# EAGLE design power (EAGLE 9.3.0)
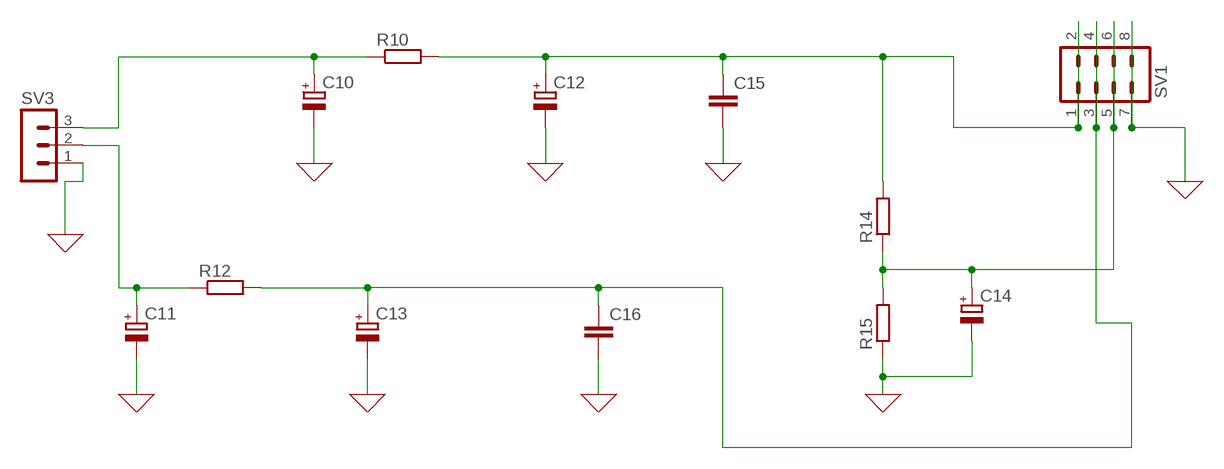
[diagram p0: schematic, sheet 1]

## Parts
C10  CPOL-EUB45181A  [B45181A]
C11  CPOL-EUB45181A  [B45181A]
C12  CPOL-EUB45181A  [B45181A]
C13  CPOL-EUB45181A  [B45181A]
C14  CPOL-EUB45181A  [B45181A]
C15  C-EUC0805  [C0805]
C16  C-EUC0805  [C0805]
R10  R-EU_M0805  [M0805]
R12  R-EU_M0805  [M0805]
R14  R-EU_M0805  [M0805]
R15  R-EU_M0805  [M0805]
SV1  MA04-2  [MA04-2]
SV3  MA03-1  [MA03-1]

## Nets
0: C10.- C11.- C12.- C13.- C14.- C15.2 C16.2 R15.1 SV1.7 SV1.8 SV3.1 ; supply symbol labelled GND
N$1: C10.+ R10.1 SV3.3
N$23: C12.+ C15.1 R10.2 R14.2 SV1.1 SV1.2
N$25: C11.+ R12.1 SV3.2
N$26: C13.+ C16.1 R12.2 SV1.3 SV1.4
N$28: C14.+ R14.1 R15.2 SV1.5 SV1.6

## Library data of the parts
C10-C14 = rcl:CPOL-EU: POLARIZED CAPACITOR, European symbol; SPICEPREFIX: C
C15 C16 = rcl:C-EU: CAPACITOR, European symbol; SPICEPREFIX: C
R10 R12 R14 R15 = rcl:R-EU_: RESISTOR, European symbol; SPICEPREFIX: R
SV1 = con-lstb:MA04-2: PIN HEADER; OC_FARNELL: unknown; OC_NEWARK: unknown
SV3 = con-lstb:MA03-1: PIN HEADER; OC_FARNELL: unknown; OC_NEWARK: unknown

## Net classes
0 default: width 0.305 mm, drill 0.406 mm, clearance 0.508 mm

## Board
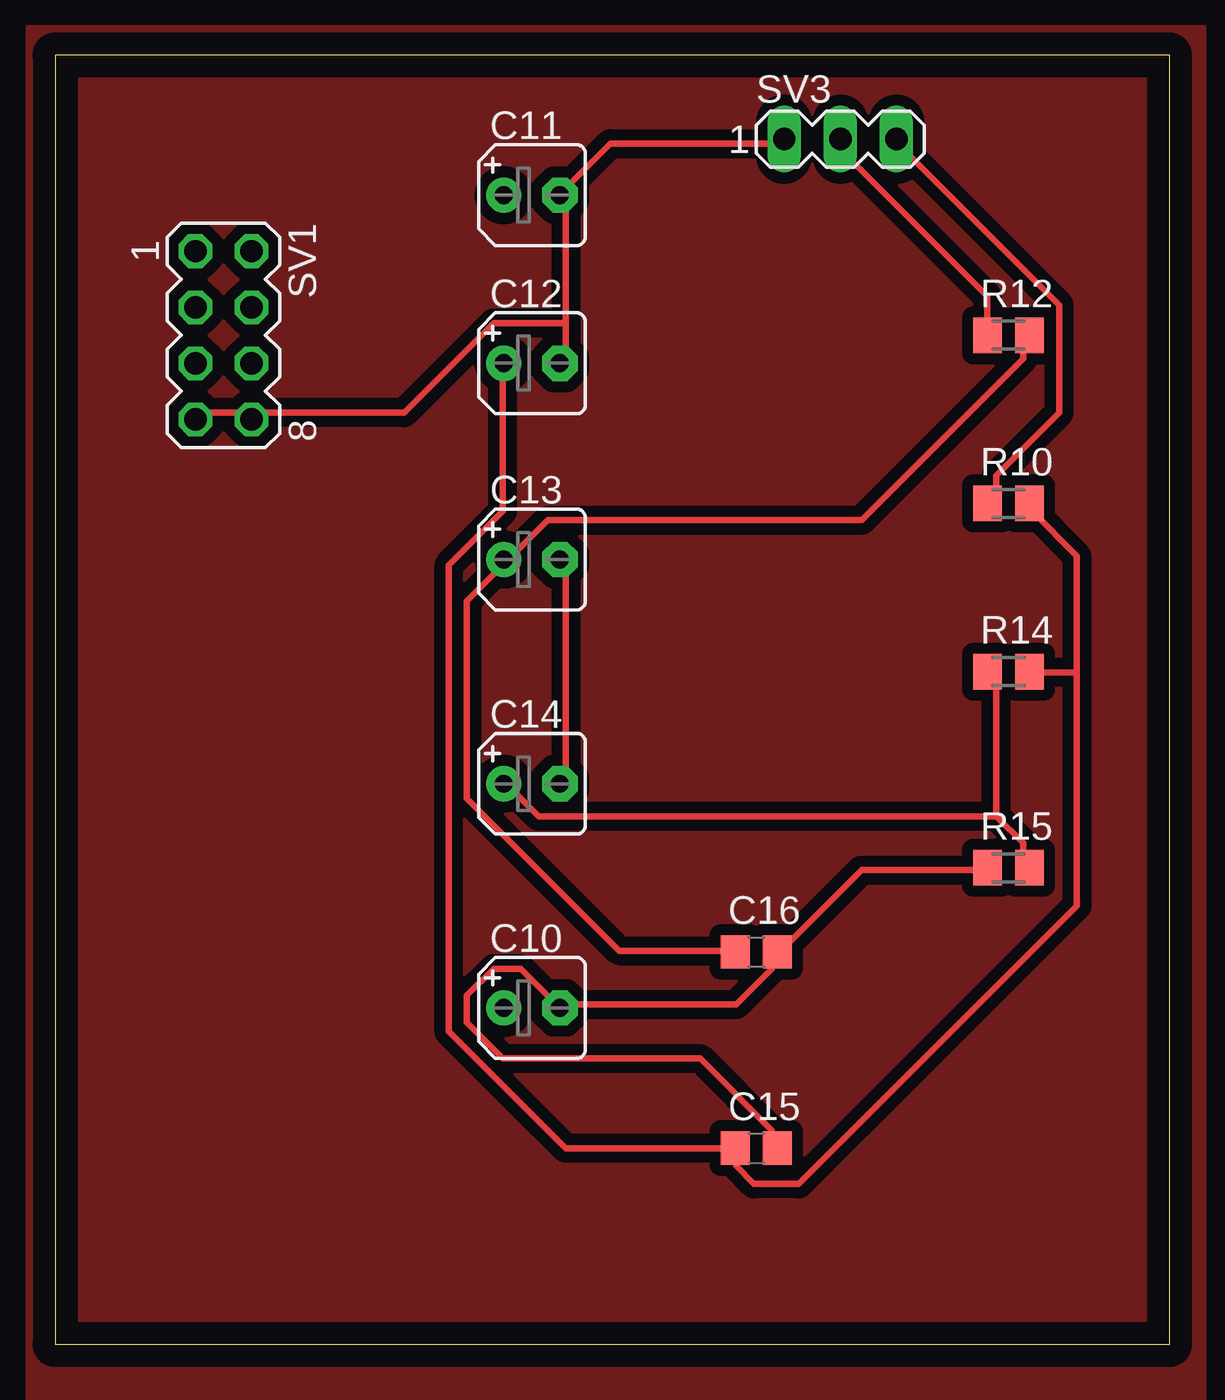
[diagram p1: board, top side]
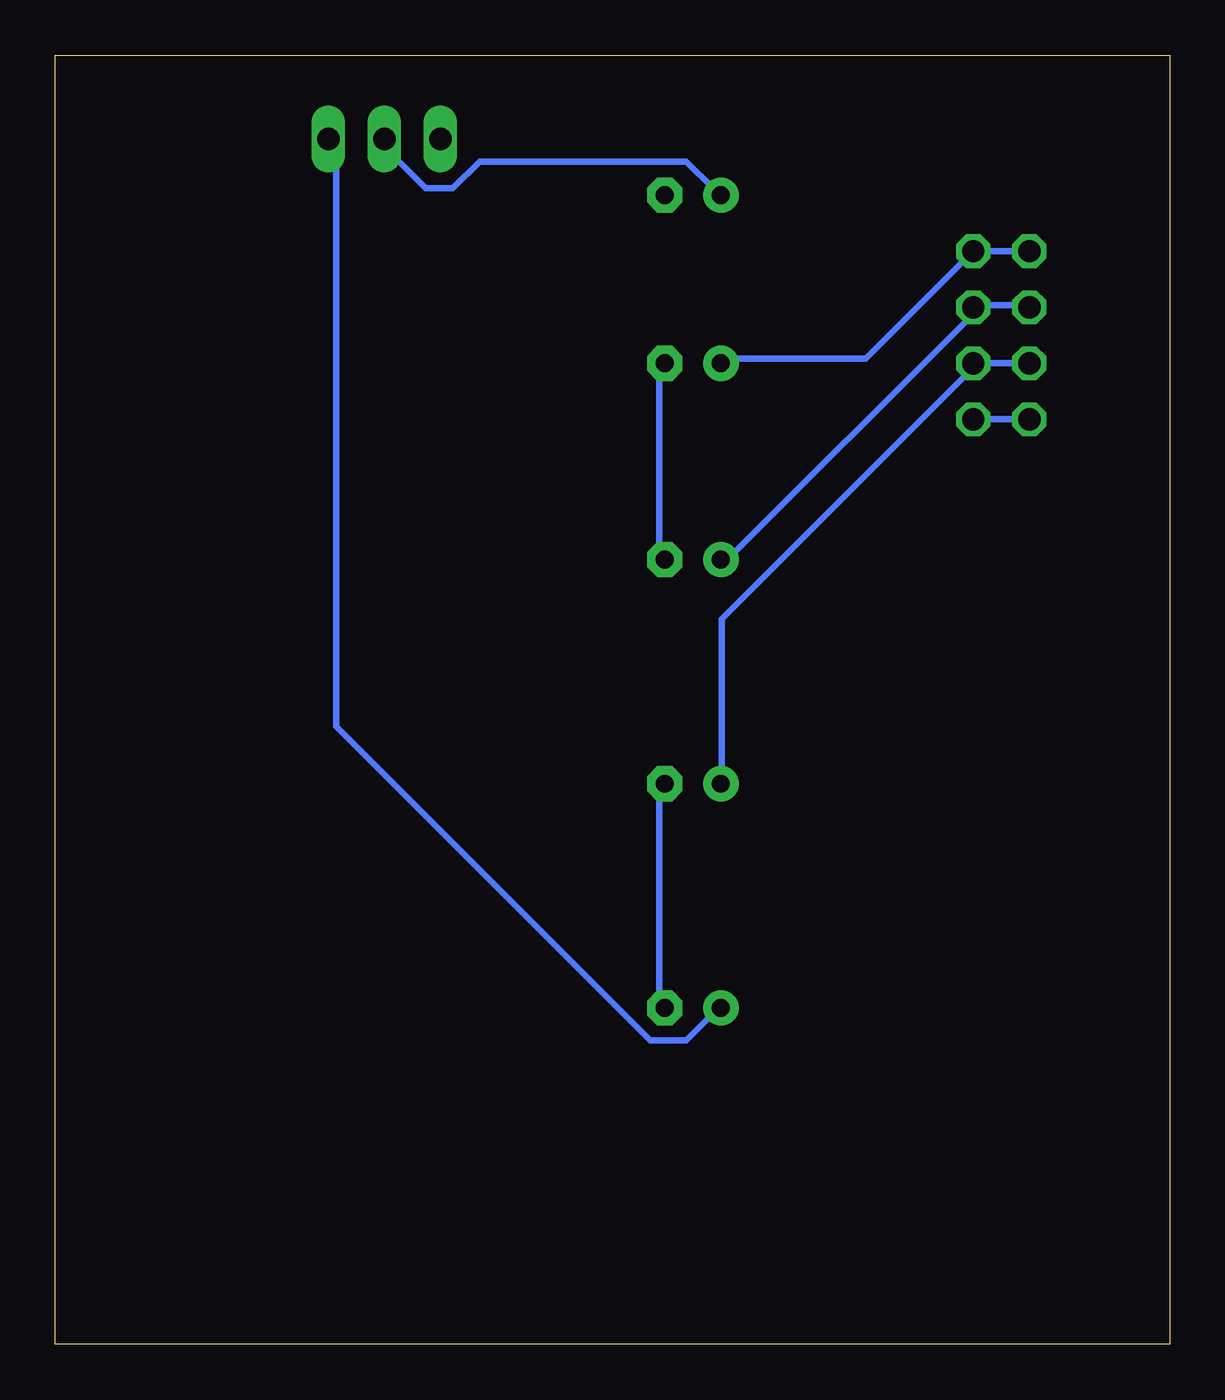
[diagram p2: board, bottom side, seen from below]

Size 50.47 x 58.41 mm. Coordinates in mm from the lower left corner, seen from the top.
Outline: 0,0 50.47,0 50.47,58.41 0,58.41 0,0
Copper layers (1*16): Top 0.035mm / dielectric 1.5mm / Bottom 0.035mm
Design rules "default": minimum track width 6mil, minimum drill 0.35mm, track to track 6mil, track to pad 6mil, pad to pad 6mil, via to via 6mil, smd to smd 6mil, copper to edge 40mil, drill to drill 6mil, minimum pad ring 10mil, minimum via ring 8mil, stop-mask expansion 4mil, vias tented up to drill 0mil, thermal gap 10mil

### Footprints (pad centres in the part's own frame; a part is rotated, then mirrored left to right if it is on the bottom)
B45181A = drill 0.813 pad 1.6: + -1.27,0 | drill 0.813 pad 1.6 octagon: - 1.27,0
C0805 = smd 1.3 x 1.5: 1 -0.95,0; 2 0.95,0
M0805 = smd 1.3 x 1.6: 1 -0.95,0; 2 0.95,0
MA04-2 = drill 1.016 octagon: 1 -3.81,-1.27; 2 -3.81,1.27; 3 -1.27,-1.27; 4 -1.27,1.27; 5 1.27,-1.27; 6 1.27,1.27; 7 3.81,-1.27; 8 3.81,1.27
MA03-1 = drill 1.016 long: 1 -2.54,0; 2 0,0; 3 2.54,0

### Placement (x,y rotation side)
C10  21.59,15.24 0 top
C11  21.59,52.07 0 top
C12  21.59,44.45 0 top
C13  21.59,35.56 0 top
C14  21.59,25.4 0 top
C15  31.75,8.89 0 top
C16  31.75,17.78 0 top
R10  43.18,38.1 0 top
R12  43.18,45.72 0 top
R14  43.18,30.48 0 top
R15  43.18,21.59 0 top
SV1  7.62,45.72 270 top
SV3  35.56,54.61 0 top

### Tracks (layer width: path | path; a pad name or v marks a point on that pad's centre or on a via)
0
  Top 0.305: C15.2 32.46,8.89 32.46,9.7 29.21,12.95 20.27,12.95 18.64,14.58 18.64,15.8 19.86,17.02 21.08,17.02 C10.- 23.11,15.39 30.84,15.39 32.46,17.02 32.46,17.42 C16.2 32.87,17.83 36.52,21.49 42.22,21.49 R15.1 | C14.- 23.11,25.55 23.11,35.31 C13.- | 8.89,42.22 6.45,42.22 SV1.7 | SV3.1 32.87,54.41 25.15,54.41 23.11,52.38 C11.- 23.11,51.97 23.11,46.28 | 23.11,46.28 23.11,44.65 C12.- | 8.89,42.22 15.8,42.22 19.86,46.28 23.11,46.28 | 8.89,42.22 SV1.8
  Bottom 0.305: C13.- 23.11,35.71 23.11,44.25 C12.- | C10.- 23.11,15.39 23.11,25.15 C14.- | SV1.8 SV1.7
GND
  pour Top: -1.27,59.69 -1.27,-2.54 52.07,-2.54 52.07,59.69
N$1
  Top 0.305: SV3.3 38.15,54.41 45.47,47.09 45.47,42.22 42.62,39.37 42.62,38.15 R10.1
  Bottom 0.305: C10.+ 20.68,14.99 21.9,13.77 23.52,13.77 37.74,27.99 37.74,54.41 SV3.3
N$23
  Top 0.305: 46.28,30.43 46.28,35.71 44.25,37.74 R10.2 | 46.28,30.43 46.28,19.86 33.68,7.26 31.65,7.26 30.84,8.08 30.84,8.89 C15.1 23.11,8.89 17.83,14.17 17.83,35.31 20.27,37.74 20.27,44.25 C12.+ | 46.28,30.43 44.25,30.43 R14.2
  Bottom 0.305: SV1.1 SV1.2 13.77,44.65 20.27,44.65 C12.+
N$25
  Top 0.305: R12.1 42.22,45.87 42.22,47.5 35.31,54.41 SV3.2
  Bottom 0.305: C11.+ 20.68,52.38 21.9,53.59 31.24,53.59 32.46,52.38 33.68,52.38 35.71,54.41 SV3.2
N$26
  Top 0.305: C16.1 30.43,17.83 25.55,17.83 18.64,24.74 18.64,33.68 20.27,35.31 C13.+ 20.68,35.71 22.3,37.34 36.52,37.34 43.84,44.65 43.84,45.47 R12.2
  Bottom 0.305: SV1.3 6.45,47.09 8.89,47.09 SV1.4 8.89,46.69 20.27,35.31 C13.+
N$28
  Top 0.305: 42.62,23.93 42.62,30.43 R14.1 | 42.62,23.93 43.84,22.71 43.84,21.89 R15.2 | 42.62,23.93 21.9,23.93 20.68,25.15 C14.+
  Bottom 0.305: C14.+ 20.27,25.55 20.27,32.87 8.89,44.25 SV1.6 SV1.5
